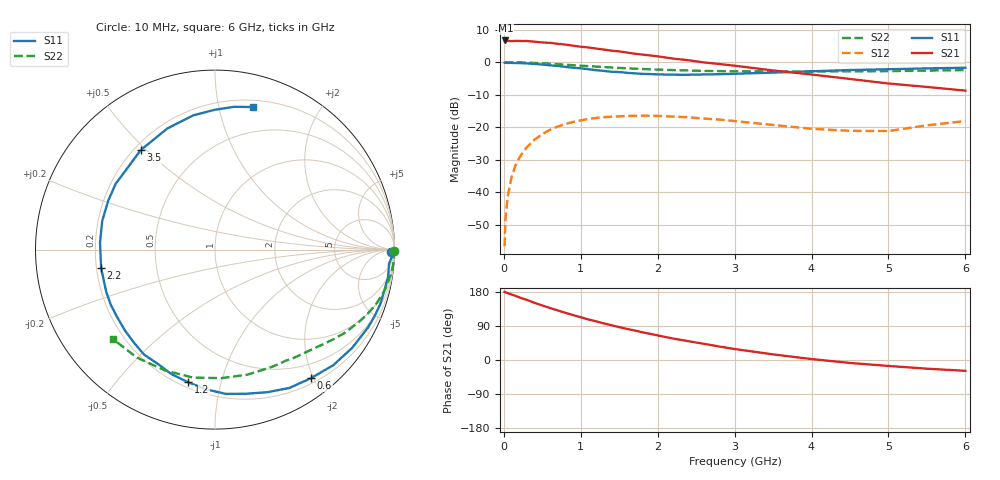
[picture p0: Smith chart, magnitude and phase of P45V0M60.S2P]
! SIEMENS Small Signal Semiconductors
! BFP182
! Si NPN RF Bipolar Junction Transistor in SOT143
! VCE = 5 V  IC = 0.6 mA
! Common Emitter S-Parameters:  March  1996
# GHz  S  MA  R  50
!  f  S11  S21  S12  S22
! GHz  MAG  ANG  MAG  ANG  MAG  ANG  MAG  ANG
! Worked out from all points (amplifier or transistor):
!   36 points, 10 MHz to 6 GHz, reference 50 ohm
!   highest |S21| = 6.7 dB at 20 MHz (marker M1)
!   |S21| within 3 dB of that: start of sweep to 1.361 GHz
!   unconditionally stable (mu >= 1): 2.883 GHz to end of sweep
!   at 250 MHz: K = 0.09, MSG = 17.0 dB, |S12| = -27.6 dB
!   at 1.4 GHz: K = 0.50, MSG = 10.1 dB, |S12| = -16.7 dB
!   at 6 GHz: K = 1.15, MAG = 2.3 dB, |S12| = -18.1 dB
!   S11 on the Smith chart (normalised r, x): 10 MHz: 68, -49; 600 MHz: 0.28, -1.97; 1.2 GHz: 0.23, -0.79; 2.2 GHz: 0.22, -0.08; 3.5 GHz: 0.23, +0.48; 6 GHz: 0.26, +1.27
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0.01  0.9807 -0.8  2.11 179.6  0.0015 80.1  0.9988 -0.3
0.02  0.9875 -2.1  2.156 179.1  0.0038 90.8  0.9921 -0.6
0.05  0.9728 -4.7  2.129 176.3  0.0086 89.3  0.9983 -1.6
0.1  0.9763 -8.9  2.105 172.9  0.0171 83.9  0.9961 -3.2
0.15  0.971 -13.6  2.121 169.2  0.0258 80.8  0.9955 -4.9
0.3  0.9568 -26.9  2.116 158.7  0.0497 72.0  0.9833 -9.8
0.4  0.9403 -35.5  2.063 150.8  0.0649 66.8  0.974 -12.9
0.6  0.894 -53.2  1.983 137.2  0.0918 55.5  0.9471 -18.7
0.8  0.847 -69.7  1.865 124.5  0.1124 45.7  0.9152 -24.0
1.1  0.7798 -93.8  1.683 107.0  0.1346 32.8  0.8694 -30.8
1.2  0.7542 -101.4  1.62 101.9  0.1394 28.4  0.8564 -33.1
1.4  0.7128 -116.2  1.503 91.6  0.1456 21.3  0.8292 -36.9
1.6  0.6871 -131.3  1.407 82.1  0.1497 15.3  0.8068 -40.4
1.9  0.6572 -152.0  1.269 69.2  0.1505 7.0  0.7778 -45.5
2.2  0.6426 -170.9  1.136 56.7  0.1463 0.3  0.7562 -50.6
2.8  0.6541 155.5  0.938 35.6  0.1315 -9.6  0.7298 -61.2
3.5  0.6918 126.7  0.747 14.8  0.1088 -13.9  0.7198 -75.5
4  0.7252 111.5  0.647 2.5  0.095 -10.1  0.717 -87.2
4.5  0.7577 99.2  0.553 -7.8  0.0883 -3.4  0.7238 -99.8
5  0.7793 90.0  0.471 -15.7  0.0878 9.6  0.7286 -112.7
5.5  0.803 82.3  0.417 -22.9  0.1075 15.1  0.7426 -126.0
6  0.8226 74.9  0.366 -28.6  0.125 16.0  0.7563 -138.8
